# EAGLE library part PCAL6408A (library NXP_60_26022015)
Low-voltage translating, 8-bit I2C-bus/SMBus I/O expander with interrupt output, reset, and configuration registers The PCAL6408A is an 8-bit general purpose I/O expander that provides remote I/O expansion for most microcontroller families via the I2C-bus interface. AAL Eindhoven MK
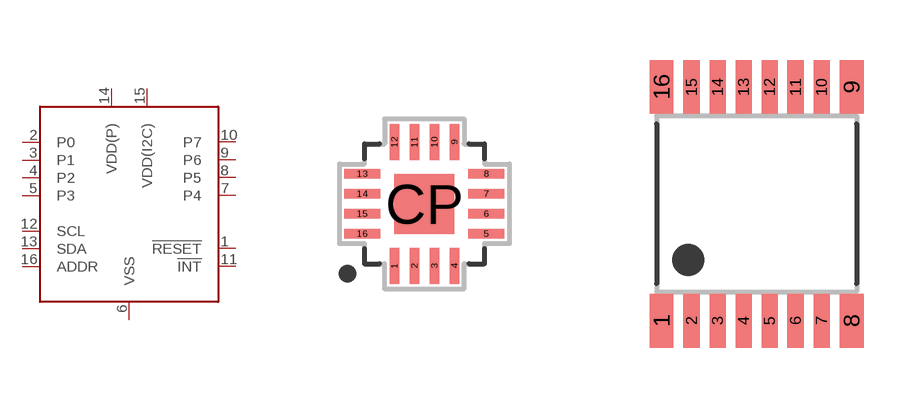
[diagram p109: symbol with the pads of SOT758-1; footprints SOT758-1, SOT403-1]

Designator prefix U

## PCAL6408ABS  [SOT758-1]
1  !RESET!  in
2  P0
3  P1
4  P2
5  P3
6  VSS
7  P4
8  P5
9  P6
10  P7
11  !INT!  out
12  SCL
13  SDA
14  VDD(P)  pwr
15  VDD(I2C)  pwr
16  ADDR  in

## PCAL6408APW  [SOT403-1]
1  VDD(I2C)  pwr
2  ADDR  in
3  !RESET!  in
4  P0
5  P1
6  P2
7  P3
8  VSS
9  P4
10  P5
11  P6
12  P7
13  !INT!  out
14  SCL
15  SDA
16  VDD(P)  pwr

## PCAL6408AHK  [SOT1161-1]
Pads as for SOT758-1

## Footprint SOT758-1 (pad centres in mm)
SOT758-1 HVQFN16: plastic thermal enhanced very thin quad flat package; no leads; 16 terminals; body 3 x 3 x 0.85 mm JEDEC: MO-220 IEC: -- JEITA: --
smd 0.24 x 0.9: 1 -0.75,-1.55; 2 -0.25,-1.55; 3 0.25,-1.55; 4 0.75,-1.55; 9 0.75,1.55; 10 0.25,1.55; 11 -0.25,1.55; 12 -0.75,1.55
smd 0.9 x 0.24: 5 1.55,-0.75; 6 1.55,-0.25; 7 1.55,0.25; 8 1.55,0.75; 13 -1.55,0.75; 14 -1.55,0.25; 15 -1.55,-0.25; 16 -1.55,-0.75
smd 1.5 x 1.5: CP 0,0

## Footprint SOT403-1 (pad centres in mm)
SOT403-1 TSSOP16: plastic thin shrink small outline package; 16 leads; body width 4.4 mm JEDEC: MO-153 IEC: ---
smd 0.6 x 1.35: 1 -2.375,-2.925; 8 2.375,-2.925; 9 2.375,2.925; 16 -2.375,2.925
smd 0.4 x 1.35: 2 -1.625,-2.925; 3 -0.975,-2.925; 4 -0.325,-2.925; 5 0.325,-2.925; 6 0.975,-2.925; 7 1.625,-2.925; 10 1.625,2.925; 11 0.975,2.925; 12 0.325,2.925; 13 -0.325,2.925; 14 -0.975,2.925; 15 -1.625,2.925

## Footprint SOT1161-1 (pad centres in mm)
SOT1161-1 XQFN16: plastic, extremely thin quad flat package; no leads;16 terminals; body 1.80 x 2.60 x 0.50 mm JEDEC: -- IEC: --
smd 0.65 x 0.22: 1 -0.725,0.6
smd 0.55 x 0.22: 2 -0.775,0.2; 3 -0.775,-0.2; 4 -0.775,-0.6; 9 0.775,-0.6; 10 0.775,-0.2; 11 0.775,0.2; 12 0.775,0.6
smd 0.22 x 0.55: 5 -0.6,-1.175; 6 -0.2,-1.175; 7 0.2,-1.175; 8 0.6,-1.175; 13 0.6,1.175; 14 0.2,1.175; 15 -0.2,1.175; 16 -0.6,1.175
